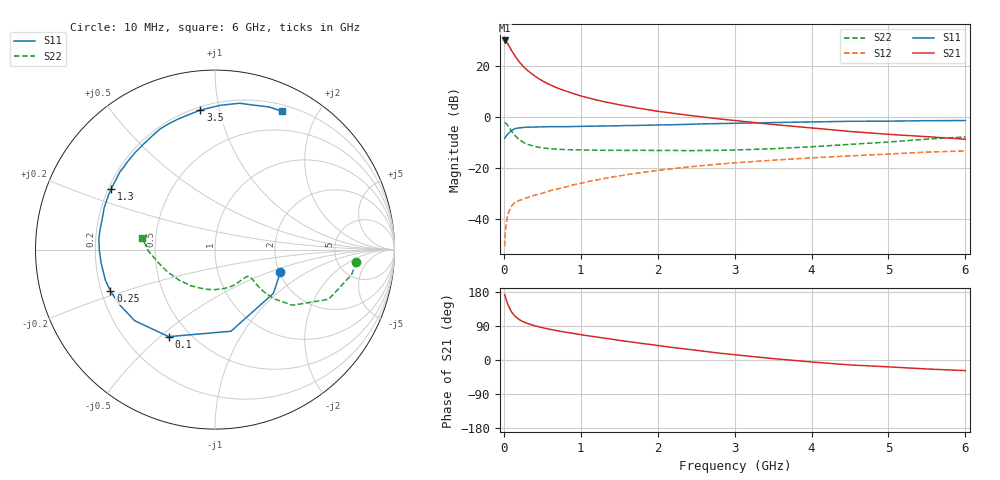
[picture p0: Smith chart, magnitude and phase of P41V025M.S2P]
! SIEMENS Small Signal Semiconductors
! BFP182
! Si NPN RF Bipolar Junction Transistor in SOT143
! VCE = 1 V  IC = 25 mA
! Common Emitter S-Parameters:  March  1996
# GHz  S  MA  R  50
!  f  S11  S21  S12  S22
! GHz  MAG  ANG  MAG  ANG  MAG  ANG  MAG  ANG
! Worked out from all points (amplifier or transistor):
!   36 points, 10 MHz to 6 GHz, reference 50 ohm
!   highest |S21| = 30.0 dB at 10 MHz (marker M1)
!   |S21| within 3 dB of that: start of sweep to 83.06 MHz
!   unconditionally stable (mu >= 1): start of sweep to 18.53 MHz; 236.8 MHz to end of sweep
!   at 250 MHz: K = 1.04, MAG = 24.8 dB, |S12| = -32.0 dB
!   at 1.4 GHz: K = 2.00, MAG = 8.7 dB, |S12| = -23.5 dB
!   at 6 GHz: K = 1.53, MAG = -2.0 dB, |S12| = -13.2 dB
!   S11 on the Smith chart (normalised r, x): 10 MHz: 2.03, -0.60; 100 MHz: 0.38, -0.53; 250 MHz: 0.24, -0.18; 1.3 GHz: 0.21, +0.26; 3.5 GHz: 0.22, +0.88; 6 GHz: 0.27, +1.56
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0.01  0.3852 -19.0  31.45 172.9  0.003 74.2  0.7902 -5.0
0.02  0.4066 -36.8  31.03 166.2  0.0058 73.2  0.7737 -10.4
0.05  0.4634 -78.9  27.36 147.4  0.0126 65.4  0.6912 -23.6
0.1  0.5493 -118.0  20.04 126.7  0.0183 47.8  0.5312 -35.7
0.15  0.5975 -138.4  15.23 114.6  0.0219 42.1  0.4268 -39.9
0.2  0.6143 -150.1  12.04 106.8  0.0234 40.4  0.3636 -40.8
0.25  0.6267 -158.4  9.846 101.1  0.025 40.5  0.3223 -40.5
0.3  0.6341 -164.4  8.352 97.0  0.0266 41.7  0.2963 -39.8
0.4  0.6389 -173.2  6.373 90.3  0.0297 44.1  0.2668 -38.5
0.5  0.6442 -179.7  5.098 85.3  0.0325 46.6  0.2504 -38.0
0.6  0.6498 175.0  4.291 81.0  0.0363 48.4  0.2409 -38.5
0.7  0.6501 170.5  3.67 77.1  0.0394 50.4  0.2354 -39.4
0.9  0.6531 163.1  2.895 70.4  0.0473 52.4  0.2294 -42.2
1.1  0.6624 155.9  2.364 63.7  0.0551 53.4  0.2266 -46.4
1.3  0.6702 149.8  2.003 57.8  0.0629 53.0  0.2242 -51.1
1.7  0.6856 137.8  1.54 46.3  0.0787 52.2  0.2235 -61.2
2.2  0.709 124.5  1.187 32.9  0.0983 48.6  0.2231 -76.4
2.8  0.7474 109.9  0.92 18.1  0.1205 43.1  0.2239 -97.1
3.5  0.7818 96.0  0.717 3.7  0.1438 36.3  0.2411 -122.7
4.5  0.8269 80.5  0.524 -13.0  0.1745 26.6  0.2931 -155.1
5.5  0.8499 69.3  0.414 -23.7  0.207 17.0  0.3714 -178.8
6  0.8563 64.2  0.37 -28.0  0.218 11.4  0.4091 171.1
